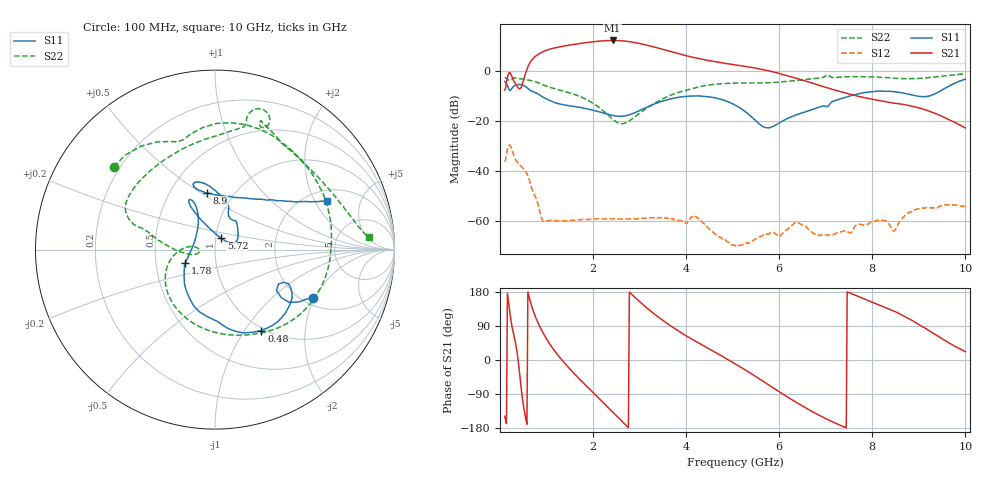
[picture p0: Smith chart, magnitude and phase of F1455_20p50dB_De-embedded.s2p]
! Integrated Device Technology
! Corporate Headquarters
! 6024 Silver Creek Valley Road
! San Jose, CA 95138  USA
! Phone:  1-408-284-8200
! Toll Free:  1-800-223-1366
! Webpage:  http://www.idt.com/
! Timing and RF Division
! 515 Groton Road, Suite 102
! Westford, MA 01886-6024
! Device:  F1455
! Description: 6-bit 0.5 dB Transmit Variable Gain Amplifier
! Frequency:  1400.0 -  2300.00 MHz
! Package:  6x6 mm Thin QFN Plastic Package: 28 pin
! State:  41
! Atten State:  20.5 dB
! Voltage:  +5.00 Volts
! Current:  217.627 mA
! Data:  The device was measured on a the F1455 evaluation board which has
!  individual transmission lines to the RF pins.  Data was collected
!  using a calibrated network analyzer.  The evaluation board was
!  de-embedded using a TRL calibration technique.
!  The reference plane is the edge of the package pin.
!  Pin  1 = CSb
!  Pin  2 = DATA
!  Pin  3 = CLK
!  Pin  4 = RSET
!  Pin  5 = GND
!  Pin  6 = RFIN  = Port 1
!  Pin  7 = GND
!  Pin  8 = NC
!  Pin  9 = NC
!  Pin 10 = NC
!  Pin 11 = NC
!  Pin 12 = NC
!  Pin 13 = NC
!  Pin 14 = /STBY
!  Pin 15 = GND
!  Pin 16 = RFOUT  = Port 2
!  Pin 17 = GND
!  Pin 18 = NC
!  Pin 19 = NC
!  Pin 20 = NC
!  Pin 21 = GND
!  Pin 22 = NC
!  Pin 23 = GND
!  Pin 24 = NC
!  Pin 25 = NC
!  Pin 26 = NC
!  Pin 27 = GND
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# GHz S dB R 50
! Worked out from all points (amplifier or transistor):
!   496 points, 100 MHz to 10 GHz, reference 50 ohm
!   highest |S21| = 12.1 dB at 2.42 GHz (marker M1)
!   |S21| within 3 dB of that: 1.176 GHz to 3.389 GHz (2.212 GHz wide, 96.9 % of centre)
!   unconditionally stable (mu >= 1): start of sweep to end of sweep
!   at 1.74 GHz: K = 119.12, MAG = 11.5 dB, |S12| = -59.6 dB
!   at 5.06 GHz: K = 792.44, MAG = 4.2 dB, |S12| = -70.0 dB
!   at 10 GHz: K = 496.87, MAG = -14.3 dB, |S12| = -54.3 dB
!   S11 on the Smith chart (normalised r, x): 100 MHz: 2.26, -1.92; 480 MHz: 0.97, -1.20; 1.78 GHz: 0.71, -0.11; 5.72 GHz: 1.06, +0.14; 8.9 GHz: 0.75, +0.53; 10 GHz: 2.47, +2.51
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0.1  -4.33 -26.2  -7.70 -148.4  -36.34 47.1  -2.76 140.7
0.26  -6.91 -24.9  -2.46 87.4  -31.83 -76.8  -3.31 95.8
0.38  -5.55 -42.0  -6.54 9.2  -36.75 -117.0  -3.05 57.9
0.48  -5.69 -60.2  -5.43 -98.7  -38.75 -148.5  -3.34 32.0
0.68  -8.12 -90.4  4.19 142.5  -46.94 139.2  -3.97 -14.3
0.82  -9.34 -108.7  6.52 97.4  -53.53 111.0  -4.80 -45.3
0.96  -10.93 -123.4  7.91 64.3  -60.51 126.6  -5.94 -70.6
1.34  -13.53 -144.7  9.76 -1.3  -60.03 100.3  -8.03 -120.9
1.76  -14.82 -155.9  11.02 -56.5  -59.49 68.6  -10.65 -157.6
1.78  -14.92 -156.3  11.07 -59.0  -59.52 66.7  -10.83 -159.1
2.1  -16.32 -166.0  11.79 -97.8  -59.21 50.4  -14.33 -179.6
2.42  -17.88 175.3  12.11 -137.1  -59.26 37.1  -19.40 172.8
2.82  -17.35 138.7  11.53 174.5  -59.32 26.2  -19.58 -167.2
3.1  -15.10 122.0  10.47 143.2  -59.16 19.3  -15.72 -172.8
3.4  -12.74 114.9  9.05 113.5  -58.75 8.5  -12.22 177.4
4.08  -10.16 116.0  5.64 58.1  -59.21 -3.3  -7.45 163.6
5.06  -13.81 116.8  2.33 -10.5  -70.04 -17.8  -4.96 148.7
5.72  -22.82 61.3  0.17 -61.5  -65.46 4.5  -4.85 121.4
6.7  -15.65 39.3  -4.91 -135.5  -64.64 -131.9  -3.24 78.7
8.36  -8.23 107.8  -12.70 134.1  -61.46 92.8  -2.84 62.7
8.9  -9.93 98.3  -14.43 100.8  -55.85 111.9  -3.18 41.3
10  -3.36 23.7  -22.92 22.1  -54.27 33.7  -1.28 4.7
